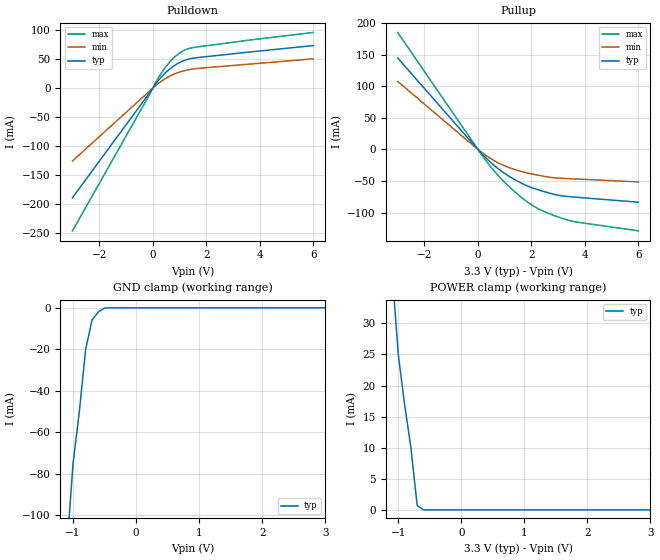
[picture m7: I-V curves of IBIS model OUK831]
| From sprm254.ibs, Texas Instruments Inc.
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[Model]   OUK831
Model_type   3-state
Polarity   Non-Inverting
Enable   Active-Low
| signals   A, GZ, Y
Cref = 20p
Rref = 50
Vmeas = 1.3
|   typ   min   max
C_comp   2.3828p   2.3362p   2.5380p
|   typ   min   max
[Temperature Range]   25.0   -40   125
|   typ   min   max
[Voltage Range]   3.3V   3.0V   3.6V
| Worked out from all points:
|   slope of the pulldown table from 0 to 0.495 V, typ, clamps not added: 18.1 ohm
|   slope of the pullup table from 0 to 0.495 V, typ, clamps not added: 23.4 ohm
|   GND clamp passes 1 mA (typ) near -0.55 V on its own axis
|   POWER clamp passes 1 mA (typ) near -0.70 V on its own axis
[Pulldown]
|   Voltage   I(typ)   I(min)   I(max)
-3V       -189.6mA   -126.1mA   -247mA
-200mV    -13.23mA   -8.458mA   -17.71mA
200mV     12.55mA    7.821mA    17.15mA
500mV     27.6mA     17.31mA    37.69mA
700mV     35.42mA    22.27mA    48.39mA
900mV     41.65mA    26.23mA    56.98mA
1.2V      48.29mA    30.47mA    66.09mA
1.5V      51.76mA    33.05mA    70.13mA
6V        73.7mA     50.67mA    96.33mA
[GND_clamp]
|   Voltage   I(typ)   I(min)   I(max)
-3V       -900mA     NA         NA
-2V       -500mA     NA         NA
-1V       -75mA      NA         NA
-900mV    -50mA      NA         NA
-800mV    -20mA      NA         NA
-700mV    -6mA       NA         NA
-600mV    -2mA       NA         NA
-500mV    -120uA     NA         NA
-400mV    0A         NA         NA
3V        0A         NA         NA
[Pullup]
|   Voltage   I(typ)   I(min)   I(max)
-3V       144.6mA    107.5mA    184.9mA
200mV     -9.093mA   -6.509mA   -12.02mA
500mV     -21.36mA   -15.05mA   -28.59mA
900mV     -35.1mA    -24.15mA   -47.86mA
1.6V      -52.84mA   -34.71mA   -75.03mA
2V        -60.26mA   -38.62mA   -87.52mA
2.3V      -64.51mA   -41.15mA   -94.69mA
2.9V      -71.54mA   -45.04mA   -105.4mA
3.4V      -74.61mA   -46.22mA   -112.3mA
6V        -83.49mA   -51.42mA   -128.8mA
[POWER_clamp]
|   Voltage   I(typ)   I(min)   I(max)
-3V       300mA      NA         NA
-2V       160mA      NA         NA
-1V       25mA       NA         NA
-900mV    17mA       NA         NA
-800mV    10mA       NA         NA
-700mV    700uA      NA         NA
-600mV    0A         NA         NA
-500mV    0A         NA         NA
3V        0A         NA         NA
[Ramp]
|   I(typ)   I(min)   I(max)
dV/dt_r   1.974/1.570n   1.772/2.430n   2.158/1.040n
dV/dt_f   1.977/1.400n   1.782/2.280n   2.159/0.920n
